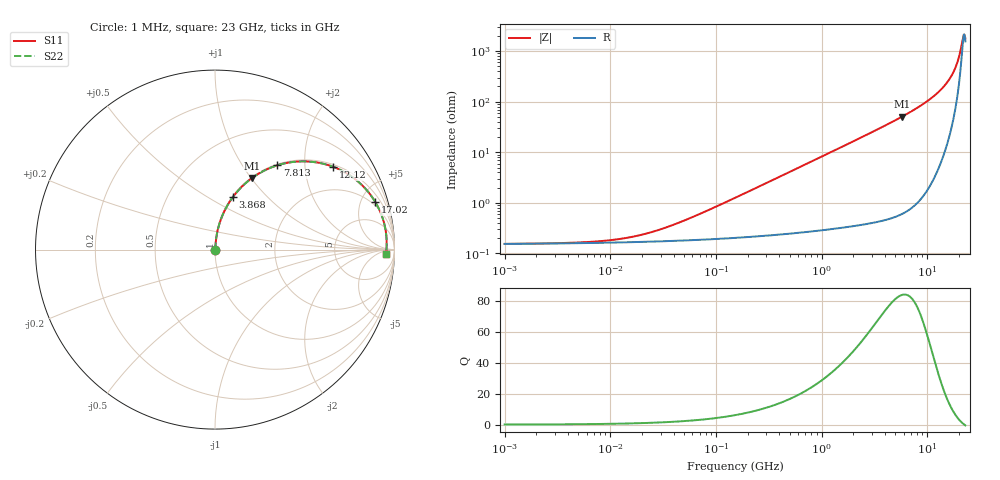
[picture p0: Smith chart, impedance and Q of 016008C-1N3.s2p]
# MHz S MA R 50
!Freq  MagS11  AngS11  MagS21  AngS21  MagS12  AngS12  MagS22  AngS22
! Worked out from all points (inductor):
!   801 points, 1 MHz to 23 GHz, reference 50 ohm
!   read as one part in series: L = 1.3 nH near 68.77 MHz
!   highest Q = 84 at 5.781 GHz (marker M1), where L = 1.39 nH
!   self-resonance near 22.43 GHz
!   S11 on the Smith chart (normalised r, x): 1 MHz: 1.00, +0.00; 3.868 GHz: 1.01, +0.65; 7.813 GHz: 1.02, +1.45; 12.12 GHz: 1.07, +2.80; 17.02 GHz: 1.62, +6.52; 23 GHz: 32, -17
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1  0.001543 3.0  0.9985 -0.0  0.9985 -0.0  0.001543 3.0
5.377611  0.001656 15.3  0.9984 -0.0  0.9984 -0.0  0.001656 15.3
13.27837  0.001977 33.1  0.9983 -0.1  0.9983 -0.1  0.001977 33.1
28.55793  0.002899 53.3  0.9983 -0.1  0.9983 -0.1  0.002899 53.3
56.25269  0.004934 68.1  0.9982 -0.3  0.9982 -0.3  0.004934 68.1
151.6575  0.01253 80.0  0.9979 -0.7  0.9979 -0.7  0.01253 80.0
815.5551  0.06643 83.8  0.9951 -3.8  0.9951 -3.8  0.06643 83.8
1891.246  0.1533 79.9  0.9848 -8.8  0.9848 -8.8  0.1533 79.9
3868.309  0.3085 71.2  0.947 -18.0  0.947 -18.0  0.3085 71.2
4331.024  0.3436 69.2  0.9347 -20.1  0.9347 -20.1  0.3436 69.2
5780.831  0.4494 62.6  0.888 -26.7  0.888 -26.7  0.4494 62.6
7813.437  0.5845 53.5  0.804 -35.8  0.804 -35.8  0.5845 53.5
9918.206  0.7041 44.3  0.6983 -44.7  0.6983 -44.7  0.7041 44.3
12124.61  0.8041 35.0  0.5737 -53.5  0.5737 -53.5  0.8041 35.0
14636.93  0.8852 25.1  0.4243 -62.1  0.4243 -62.1  0.8852 25.1
17016.73  0.932 16.5  0.2847 -68.1  0.2847 -68.1  0.932 16.5
18119.11  0.9449 12.8  0.2228 -69.4  0.2228 -69.4  0.9449 12.8
19292.9  0.9535 9.0  0.1602 -68.7  0.1602 -68.7  0.9535 9.0
20033.37  0.9565 6.7  0.1231 -66.0  0.1231 -66.0  0.9565 6.7
21600.66  0.9573 2.2  0.05728 -40.7  0.05728 -40.7  0.9573 2.2
22429.7  0.9552 -0.0  0.04482 0.1  0.04482 0.1  0.9552 -0.0
23000  0.9528 -1.5  0.05358 27.6  0.05358 27.6  0.9528 -1.5
